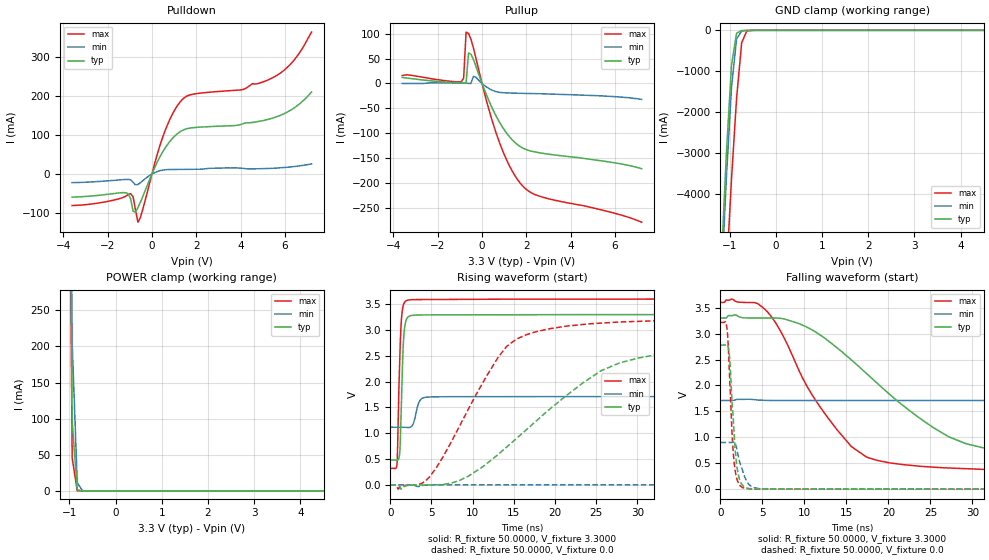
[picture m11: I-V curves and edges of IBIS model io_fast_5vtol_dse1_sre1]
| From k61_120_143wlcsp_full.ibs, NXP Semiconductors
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[Model]  io_fast_5vtol_dse1_sre1
|   Model io_fast_5vtol_dse1_sre1
| Library cells for typ/min/max conditions are connected as defined below:
|  pad - External Pad
|  ipp_do - Core Input
|  ipp_obe - Output Buffer Enable
|  esd_boost - vdd_s_3v
|  esd_bus - vdd_s_3v
|  ipp_ame - vss_s_lv
|  ipp_dse - vdd_s_lv
|  ipp_ina40a_5vtol - NC
|  ipp_ina40b_5vtol - NC
|  ipp_ina_5vtol - NC
|  ipp_ina_mux_3v - NC
|  ipp_ind - NC
|  ipp_ind_3v - NC
|  ipp_pue - vss_s_lv
|  ipp_sre - vdd_s_lv
|  tie_3v - vdd_s_3v
|  tie_hi - vdd_s_lv
|  vbuf_3v - vdd_s_3v
|  vdd_bulk_lv - vdd_s_lv
|  vdd_s_3v - vdd_s_3v
|  vdd_s_lv - vdd_s_lv
|  vss_bulk - vss_s_3v
|  vss_s_3v - vss_s_3v
|  vss_s_lv - vss_s_lv
| All other pins connected to ground
Model_type I/O
Polarity   Non-Inverting
Enable   Active-High
Vinl =   1.1550V
Vinh =   2.3100V
Vmeas =  1.6500V
Cref =   25.0000pF
Rref =   50.0000
Vref =   0.0V
C_comp   4.6092pF   4.5386pF   4.8302pF
[Temperature Range]   25.0000   0.1250k   -40.0000
[Voltage Range]   3.3000V   1.7100V   3.6000V
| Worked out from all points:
|   slope of the pulldown table from 0 to 0.495 V, typ, clamps not added: 8.59 ohm
|   slope of the pullup table from 0 to 0.495 V, typ, clamps not added: 9.33 ohm
|   GND clamp passes 1 mA (typ) near -0.54 V on its own axis
|   POWER clamp passes 1 mA (typ) near -0.79 V on its own axis
|   rising waveform, R_fixture 50.0000, V_fixture 3.3000: 20-80 % time 330ps typ, 561ps min, 337ps max; typ from 0.481 V to 3.3 V
|   rising waveform, R_fixture 50.0000, V_fixture 0.0: 20-80 % time 12.9ns typ, 76.1ns min, 6.83ns max; typ from 0 V to 2.78 V
|   falling waveform, R_fixture 50.0000, V_fixture 3.3000: 20-80 % time 13ns typ, 71.9ns min, 7.28ns max; typ from 3.3 V to 0.481 V
|   falling waveform, R_fixture 50.0000, V_fixture 0.0: 20-80 % time 660ps typ, 1.02ns min, 576ps max; typ from 2.78 V to 0 V
[Pulldown]
|Voltage   I(typ)   I(min)   I(max)
-3.6V     -59.22mA   -21.99mA   -80.5mA
-1.29V    -47.58mA   -14.27mA   -59.74mA
-960mV    -63.34mA   -14.81mA   -50.29mA
-850mV    -95.19mA   -20.91mA   -58.11mA
-630mV    -85.86mA   -26.77mA   -123.3mA
470mV     55.27mA    9.988mA    91.83mA
910mV     90.4mA     11.72mA    152.1mA
1.35V     111mA      11.98mA    189.9mA
4.1V      128.8mA    14.7mA     216.5mA
5.42V     142.9mA    14.8mA     246mA
6.41V     169.2mA    19.2mA     291.7mA
7.2V      210mA      26.1mA     363.7mA
[Pullup]
|Voltage   I(typ)   I(min)   I(max)
-3.6V     12.1mA     100uA      16mA
-940mV    1.771mA    831uA      3.465mA
-830mV    1.246mA    693.7uA    10.48mA
-720mV    725.2uA    466uA      103.4mA
-610mV    61.29mA    256uA      100.8mA
-390mV    48.58mA    14.37mA    71.55mA
270mV     -30.63mA   -9.028mA   -46.21mA
710mV     -71.72mA   -17.2mA    -109.3mA
1.26V     -108.3mA   -19.14mA   -167.8mA
1.81V     -129.2mA   -19.8mA    -205.1mA
2.69V     -140.1mA   -20.72mA   -228.1mA
7.2V      -171.4mA   -32mA      -279mA
[GND_clamp]
|Voltage   I(typ)   I(min)   I(max)
-3.6V     -73.34A    -73.38A    -74.77A
-1.18V    -5.66A     -6.204A    -8.642A
-1.07V    -2.998A    -3.591A    -5.955A
-960mV    -859.3mA   -1.396A    -3.637A
-850mV    -67.61mA   -209.6mA   -1.663A
-740mV    -7.668mA   -15.82mA   -304.8mA
-630mV    -2.587mA   -2.146mA   -18.83mA
-520mV    -662.1uA   -523uA     -1.741mA
7.2V      0A         0A         0A
[POWER_clamp]
|Voltage   I(typ)   I(min)   I(max)
-3.6V     45.85A     45.45A     46.17A
-1.05V    1.004A     1.14A      941.6mA
-940mV    96.57mA    206.1mA    45.73mA
-830mV    1.646mA    11.48mA    218.1uA
-720mV    22.84uA    474.3uA    919.1nA
-610mV    316.6nA    19.24uA    4.178nA
7.2V      0A         0A         0A
[Ramp]
| variable   typ   min   max
dV/dt_r  1.6664/12.8984n   0.5261/76.0892n   1.9284/6.8253n
dV/dt_f  1.6912/13.0232n   0.3402/71.9289n   1.9685/7.2848n
R_load = 50.0000
[Rising Waveform]
R_fixture= 50.0000
V_fixture= 3.3000
V_fixture_min= 1.7100
V_fixture_max= 3.6000
|time   V(typ)   V(min)   V(max)
0s        481.4mV    1.117V     319.2mV
804.4ps   480mV      1.117V     380.1mV
883.2ps   479.6mV    1.117V     656.5mV
1.123ns   578.1mV    1.117V     2.286V
1.34ns    1.567V     1.117V     3.188V
1.653ns   2.908V     1.117V     3.511V
2.468ns   3.278V     1.119V     3.587V
3.723ns   3.292V     1.659V     3.59V
5.7ns     3.294V     1.706V     3.591V
250ns     3.3V       1.71V      3.6V
[Rising Waveform]
R_fixture= 50.0000
V_fixture= 0.0
V_fixture_min= 0.0
V_fixture_max= 0.0
|time   V(typ)   V(min)   V(max)
0s        310.4pV    53.92nV    167.4pV
4.748ns   -2.75mV    -1.958mV   150.2mV
9.436ns   163.1mV    -376.7uV   1.455V
14.12ns   731.3mV    -382.3uV   2.684V
17.64ns   1.229V     -385.3uV   2.966V
24.04ns   2.046V     -360.3uV   3.119V
32.17ns   2.518V     298.6uV    3.179V
50.74ns   2.721V     28.4mV     3.21V
150.7ns   2.777V     700.1mV    3.214V
250ns     2.777V     876.9mV    3.214V
[Falling Waveform]
R_fixture= 50.0000
V_fixture= 3.3000
V_fixture_min= 1.7100
V_fixture_max= 3.6000
|time   V(typ)   V(min)   V(max)
0s        3.3V       1.71V      3.6V
4.061ns   3.3V       1.725V     3.597V
5.581ns   3.3V       1.711V     3.422V
10.9ns    3.072V     1.71V      1.822V
15.59ns   2.491V     1.71V      820.2mV
23.83ns   1.357V     1.71V      440.3mV
31.28ns   797.6mV    1.71V      381.5mV
50.34ns   569.8mV    1.696V     336.6mV
142ns     483mV      1.282V     319.3mV
250ns     481.4mV    1.143V     319.2mV
[Falling Waveform]
R_fixture= 50.0000
V_fixture= 0.0
V_fixture_min= 0.0
V_fixture_max= 0.0
|time   V(typ)   V(min)   V(max)
0s        2.777V     899.4mV    3.214V
599ps     2.777V     899.4mV    3.23V
807.6ps   2.788V     899.4mV    3.063V
930.9ps   2.739V     899.4mV    2.791V
1.131ns   2.464V     898.5mV    1.992V
1.442ns   1.563V     904.9mV    911.8mV
1.743ns   800.9mV    889.6mV    371mV
2.299ns   176.1mV    521.9mV    77.33mV
3.234ns   17.76mV    126.4mV    9.441mV
250ns     -258.3nV   8.418uV    -973.4pV
